FUNCTION "FC_PROG_FSH_OFF" : VOID
TITLE =FC PROG BASE FLASH-OFF
{ S7_language := '9(1) Angielski (Stany Zjednoczone)  11.01.2022  09:45:15' }
VERSION : 0.1

BEGIN
NETWORK
TITLE =

NETWORK
TITLE =Status Flash-Off ON
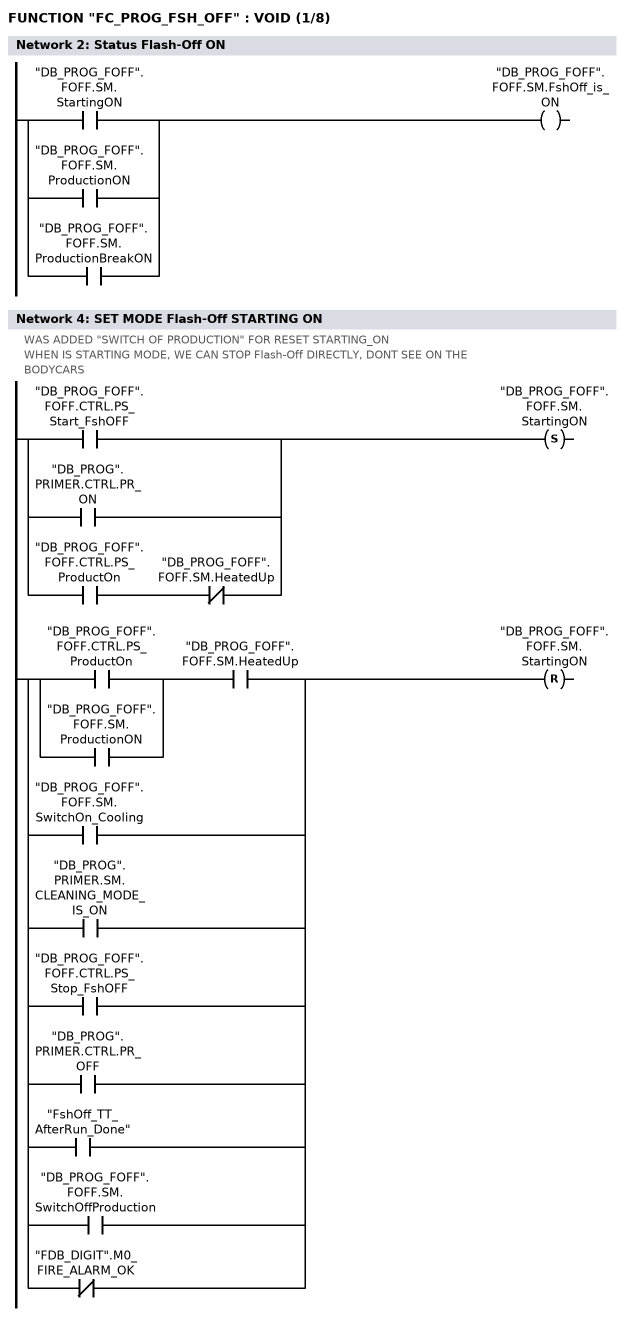
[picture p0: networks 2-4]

      O     "DB_PROG_FOFF".FOFF.SM.StartingON;
      O     "DB_PROG_FOFF".FOFF.SM.ProductionON;
      O     "DB_PROG_FOFF".FOFF.SM.ProductionBreakON;
      =     "DB_PROG_FOFF".FOFF.SM.FshOff_is_ON;
NETWORK
TITLE =SET MODE OF Flash-Off
//
//**************** SET MODE OF Flash-Off
//****************************************************
//


NETWORK
TITLE =SET MODE Flash-Off STARTING ON
//WAS ADDED "SWITCH OF PRODUCTION" FOR RESET STARTING_ON
//WHEN IS STARTING MODE, WE CAN STOP Flash-Off DIRECTLY, DONT SEE ON THE
//BODYCARS
      U(    ;
      O     "DB_PROG_FOFF".FOFF.CTRL.PS_Start_FshOFF;
      O     "DB_PROG".PRIMER.CTRL.PR_ON;
      O     ;
      U     "DB_PROG_FOFF".FOFF.CTRL.PS_ProductOn;
      UN    "DB_PROG_FOFF".FOFF.SM.HeatedUp;
      )     ;
      S     "DB_PROG_FOFF".FOFF.SM.StartingON;
      U(    ;
      U(    ;
      O     "DB_PROG_FOFF".FOFF.CTRL.PS_ProductOn;
      O     "DB_PROG_FOFF".FOFF.SM.ProductionON;
      )     ;
      U     "DB_PROG_FOFF".FOFF.SM.HeatedUp;
      O     "DB_PROG_FOFF".FOFF.SM.SwitchOn_Cooling;
      O     "DB_PROG".PRIMER.SM.CLEANING_MODE_IS_ON;
      O     "DB_PROG_FOFF".FOFF.CTRL.PS_Stop_FshOFF;
      O     "DB_PROG".PRIMER.CTRL.PR_OFF;
      O     "FshOff_TT_AfterRun_Done";
      O     "DB_PROG_FOFF".FOFF.SM.SwitchOffProduction;
      ON    "FDB_DIGIT".M0_FIRE_ALARM_OK;
      )     ;
      R     "DB_PROG_FOFF".FOFF.SM.StartingON;
      NOP   0;
NETWORK
TITLE =FLASH-OFF BASE PRODUCTION ON
//
//-----------------------------------------------------------------
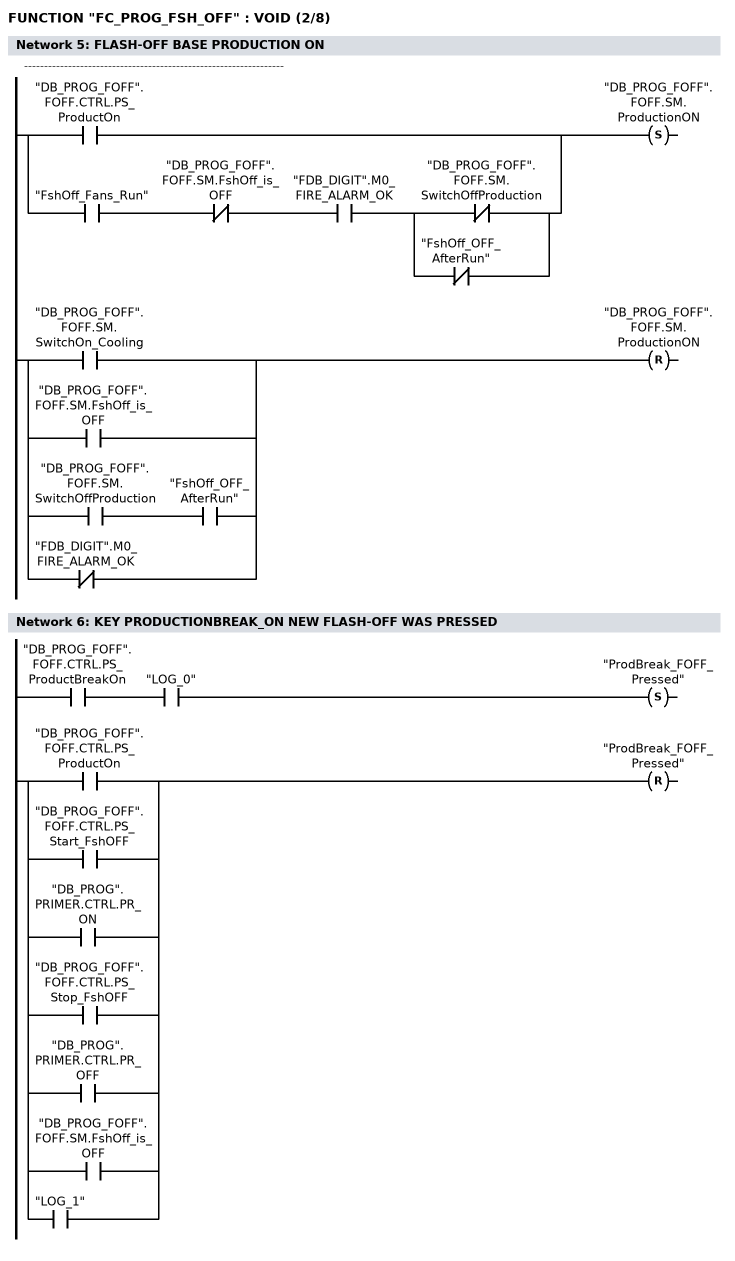
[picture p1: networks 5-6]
      U(    ;
      O     "DB_PROG_FOFF".FOFF.CTRL.PS_ProductOn;
      O     ;
      U     "FshOff_Fans_Run";
      UN    "DB_PROG_FOFF".FOFF.SM.FshOff_is_OFF;
      U     "FDB_DIGIT".M0_FIRE_ALARM_OK;
      U(    ;
      ON    "DB_PROG_FOFF".FOFF.SM.SwitchOffProduction;
      ON    "FshOff_OFF_AfterRun";
      )     ;
      )     ;
      S     "DB_PROG_FOFF".FOFF.SM.ProductionON;
      U(    ;
      O     "DB_PROG_FOFF".FOFF.SM.SwitchOn_Cooling;
      O     "DB_PROG_FOFF".FOFF.SM.FshOff_is_OFF;
      O     ;
      U     "DB_PROG_FOFF".FOFF.SM.SwitchOffProduction;
      U     "FshOff_OFF_AfterRun";
      ON    "FDB_DIGIT".M0_FIRE_ALARM_OK;
      )     ;
      R     "DB_PROG_FOFF".FOFF.SM.ProductionON;
      NOP   0;
NETWORK
TITLE =KEY PRODUCTIONBREAK_ON NEW FLASH-OFF WAS PRESSED

      U     "DB_PROG_FOFF".FOFF.CTRL.PS_ProductBreakOn;
      U     "LOG_0";
      S     "ProdBreak_FOFF_Pressed";
      U(    ;
      O     "DB_PROG_FOFF".FOFF.CTRL.PS_ProductOn;
      O     "DB_PROG_FOFF".FOFF.CTRL.PS_Start_FshOFF;
      O     "DB_PROG".PRIMER.CTRL.PR_ON;
      O     "DB_PROG_FOFF".FOFF.CTRL.PS_Stop_FshOFF;
      O     "DB_PROG".PRIMER.CTRL.PR_OFF;
      O     "DB_PROG_FOFF".FOFF.SM.FshOff_is_OFF;
      O     "LOG_1";
      )     ;
      R     "ProdBreak_FOFF_Pressed";
      NOP   0;
NETWORK
TITLE =SET MODE Flash-Off PRODUCTION BREAK ON
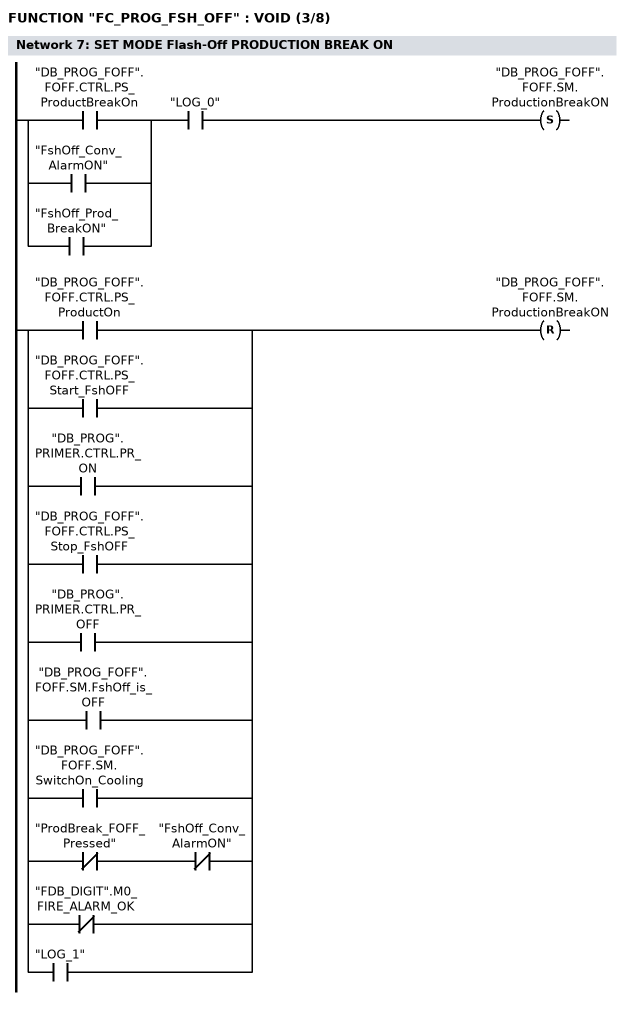
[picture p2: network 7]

      U(    ;
      O     "DB_PROG_FOFF".FOFF.CTRL.PS_ProductBreakOn;
      O     "FshOff_Conv_AlarmON";
      O     "FshOff_Prod_BreakON";
      )     ;
      U     "LOG_0";
      S     "DB_PROG_FOFF".FOFF.SM.ProductionBreakON;
      U(    ;
      O     "DB_PROG_FOFF".FOFF.CTRL.PS_ProductOn;
      O     "DB_PROG_FOFF".FOFF.CTRL.PS_Start_FshOFF;
      O     "DB_PROG".PRIMER.CTRL.PR_ON;
      O     "DB_PROG_FOFF".FOFF.CTRL.PS_Stop_FshOFF;
      O     "DB_PROG".PRIMER.CTRL.PR_OFF;
      O     "DB_PROG_FOFF".FOFF.SM.FshOff_is_OFF;
      O     "DB_PROG_FOFF".FOFF.SM.SwitchOn_Cooling;
      O     ;
      UN    "ProdBreak_FOFF_Pressed";
      UN    "FshOff_Conv_AlarmON";
      ON    "FDB_DIGIT".M0_FIRE_ALARM_OK;
      O     "LOG_1";
      )     ;
      R     "DB_PROG_FOFF".FOFF.SM.ProductionBreakON;
      NOP   0;
NETWORK
TITLE =SET MODE Flash-Off OFF
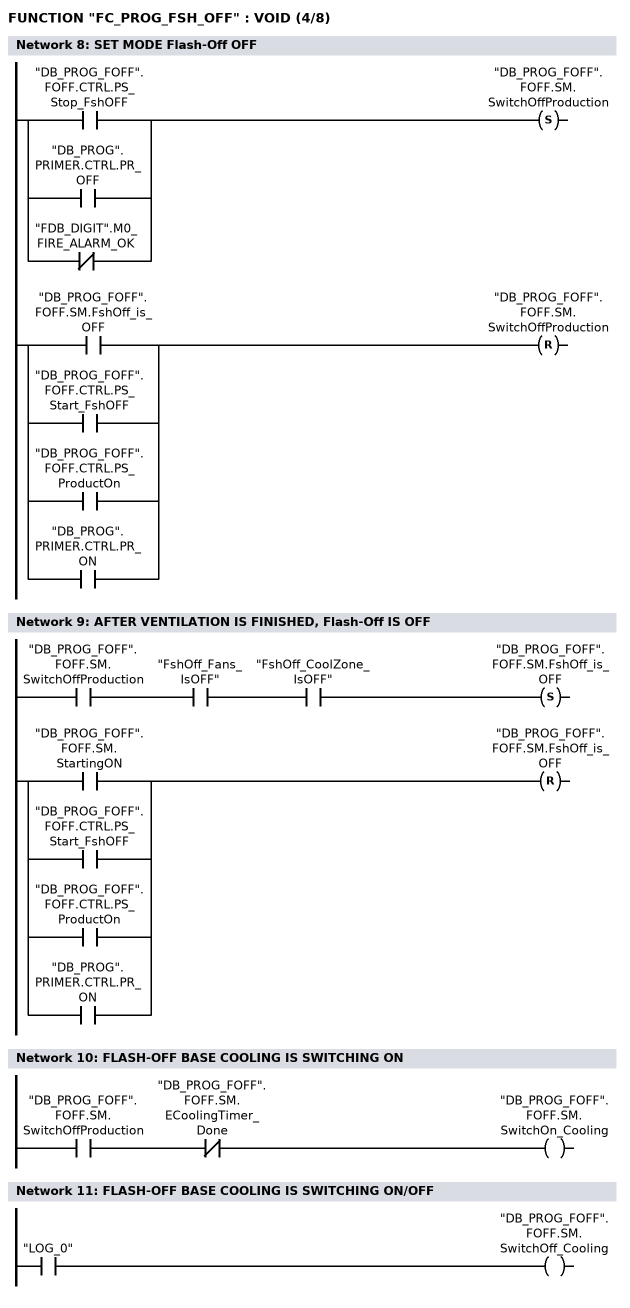
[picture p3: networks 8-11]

      U(    ;
      O     "DB_PROG_FOFF".FOFF.CTRL.PS_Stop_FshOFF;
      O     "DB_PROG".PRIMER.CTRL.PR_OFF;
      ON    "FDB_DIGIT".M0_FIRE_ALARM_OK;
      )     ;
      S     "DB_PROG_FOFF".FOFF.SM.SwitchOffProduction;
      U(    ;
      O     "DB_PROG_FOFF".FOFF.SM.FshOff_is_OFF;
      O     "DB_PROG_FOFF".FOFF.CTRL.PS_Start_FshOFF;
      O     "DB_PROG_FOFF".FOFF.CTRL.PS_ProductOn;
      O     "DB_PROG".PRIMER.CTRL.PR_ON;
      )     ;
      R     "DB_PROG_FOFF".FOFF.SM.SwitchOffProduction;
      NOP   0;
NETWORK
TITLE =AFTER VENTILATION IS FINISHED, Flash-Off IS OFF

      U     "DB_PROG_FOFF".FOFF.SM.SwitchOffProduction;
      U     "FshOff_Fans_IsOFF";
      U     "FshOff_CoolZone_IsOFF";
      S     "DB_PROG_FOFF".FOFF.SM.FshOff_is_OFF;
      U(    ;
      O     "DB_PROG_FOFF".FOFF.SM.StartingON;
      O     "DB_PROG_FOFF".FOFF.CTRL.PS_Start_FshOFF;
      O     "DB_PROG_FOFF".FOFF.CTRL.PS_ProductOn;
      O     "DB_PROG".PRIMER.CTRL.PR_ON;
      )     ;
      R     "DB_PROG_FOFF".FOFF.SM.FshOff_is_OFF;
      NOP   0;
NETWORK
TITLE =FLASH-OFF BASE COOLING IS SWITCHING ON

      U     "DB_PROG_FOFF".FOFF.SM.SwitchOffProduction;
      UN    "DB_PROG_FOFF".FOFF.SM.ECoolingTimer_Done;
      =     "DB_PROG_FOFF".FOFF.SM.SwitchOn_Cooling;
NETWORK
TITLE =FLASH-OFF BASE COOLING IS SWITCHING ON/OFF

      U     "LOG_0";
      =     "DB_PROG_FOFF".FOFF.SM.SwitchOff_Cooling;
NETWORK
TITLE =EMERGENCY COOLING ON
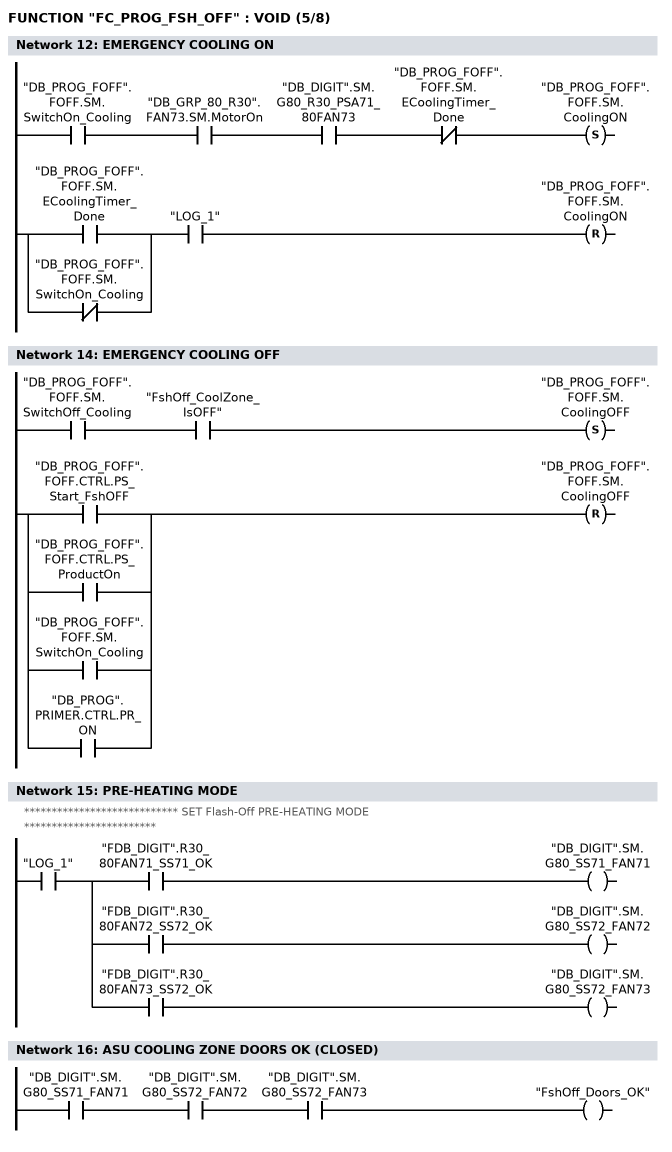
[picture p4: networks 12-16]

      U     "DB_PROG_FOFF".FOFF.SM.SwitchOn_Cooling;
      U     "DB_GRP_80_R30".FAN73.SM.MotorOn;
      U     "DB_DIGIT".SM.G80_R30_PSA71_80FAN73;
      UN    "DB_PROG_FOFF".FOFF.SM.ECoolingTimer_Done;
      S     "DB_PROG_FOFF".FOFF.SM.CoolingON;
      U(    ;
      O     "DB_PROG_FOFF".FOFF.SM.ECoolingTimer_Done;
      ON    "DB_PROG_FOFF".FOFF.SM.SwitchOn_Cooling;
      )     ;
      U     "LOG_1";
      R     "DB_PROG_FOFF".FOFF.SM.CoolingON;
      NOP   0;
NETWORK
TITLE =

NETWORK
TITLE =EMERGENCY COOLING OFF

      U     "DB_PROG_FOFF".FOFF.SM.SwitchOff_Cooling;
      U     "FshOff_CoolZone_IsOFF";
      S     "DB_PROG_FOFF".FOFF.SM.CoolingOFF;
      U(    ;
      O     "DB_PROG_FOFF".FOFF.CTRL.PS_Start_FshOFF;
      O     "DB_PROG_FOFF".FOFF.CTRL.PS_ProductOn;
      O     "DB_PROG_FOFF".FOFF.SM.SwitchOn_Cooling;
      O     "DB_PROG".PRIMER.CTRL.PR_ON;
      )     ;
      R     "DB_PROG_FOFF".FOFF.SM.CoolingOFF;
      NOP   0;
NETWORK
TITLE =PRE-HEATING MODE
//
//**************************** SET Flash-Off PRE-HEATING MODE
//************************
//


      U     "LOG_1";
      =     L      0.0;
      U     L      0.0;
      U     "FDB_DIGIT".R30_80FAN71_SS71_OK;
      =     "DB_DIGIT".SM.G80_SS71_FAN71;
      U     L      0.0;
      U     "FDB_DIGIT".R30_80FAN72_SS72_OK;
      =     "DB_DIGIT".SM.G80_SS72_FAN72;
      U     L      0.0;
      U     "FDB_DIGIT".R30_80FAN73_SS72_OK;
      =     "DB_DIGIT".SM.G80_SS72_FAN73;
NETWORK
TITLE =ASU COOLING ZONE DOORS OK (CLOSED)

      U     "DB_DIGIT".SM.G80_SS71_FAN71;
      U     "DB_DIGIT".SM.G80_SS72_FAN72;
      U     "DB_DIGIT".SM.G80_SS72_FAN73;
      =     "FshOff_Doors_OK";
NETWORK
TITLE =Flash-Off CHAIN ON
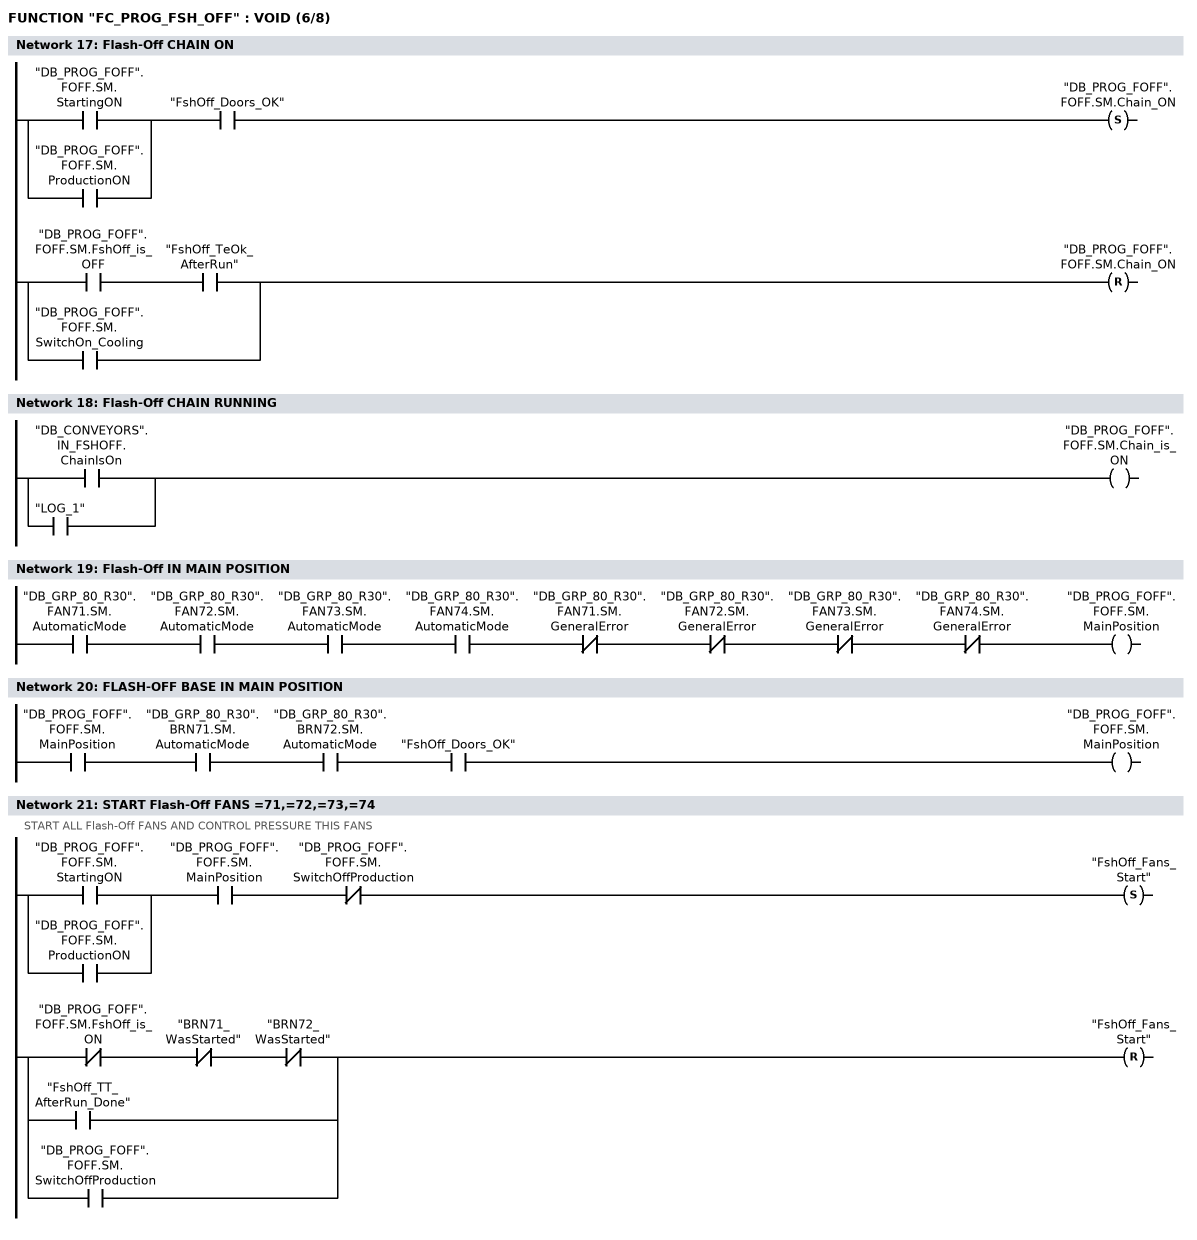
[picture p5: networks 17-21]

      U(    ;
      O     "DB_PROG_FOFF".FOFF.SM.StartingON;
      O     "DB_PROG_FOFF".FOFF.SM.ProductionON;
      )     ;
      U     "FshOff_Doors_OK";
      S     "DB_PROG_FOFF".FOFF.SM.Chain_ON;
      U(    ;
      U     "DB_PROG_FOFF".FOFF.SM.FshOff_is_OFF;
      U     "FshOff_TeOk_AfterRun";
      O     "DB_PROG_FOFF".FOFF.SM.SwitchOn_Cooling;
      )     ;
      R     "DB_PROG_FOFF".FOFF.SM.Chain_ON;
      NOP   0;
NETWORK
TITLE =Flash-Off CHAIN RUNNING

      O     "DB_CONVEYORS".IN_FSHOFF.ChainIsOn;
      O     "LOG_1";
      =     "DB_PROG_FOFF".FOFF.SM.Chain_is_ON;
NETWORK
TITLE =Flash-Off IN MAIN POSITION

      U     "DB_GRP_80_R30".FAN71.SM.AutomaticMode;
      U     "DB_GRP_80_R30".FAN72.SM.AutomaticMode;
      U     "DB_GRP_80_R30".FAN73.SM.AutomaticMode;
      U     "DB_GRP_80_R30".FAN74.SM.AutomaticMode;
      UN    "DB_GRP_80_R30".FAN71.SM.GeneralError;
      UN    "DB_GRP_80_R30".FAN72.SM.GeneralError;
      UN    "DB_GRP_80_R30".FAN73.SM.GeneralError;
      UN    "DB_GRP_80_R30".FAN74.SM.GeneralError;
      =     "DB_PROG_FOFF".FOFF.SM.MainPosition;
NETWORK
TITLE =FLASH-OFF BASE IN MAIN POSITION

      U     "DB_PROG_FOFF".FOFF.SM.MainPosition;
      U     "DB_GRP_80_R30".BRN71.SM.AutomaticMode;
      U     "DB_GRP_80_R30".BRN72.SM.AutomaticMode;
      U     "FshOff_Doors_OK";
      =     "DB_PROG_FOFF".FOFF.SM.MainPosition;
NETWORK
TITLE =START Flash-Off FANS =71,=72,=73,=74
//START ALL Flash-Off FANS AND CONTROL PRESSURE THIS FANS
//
//
      U(    ;
      O     "DB_PROG_FOFF".FOFF.SM.StartingON;
      O     "DB_PROG_FOFF".FOFF.SM.ProductionON;
      )     ;
      U     "DB_PROG_FOFF".FOFF.SM.MainPosition;
      UN    "DB_PROG_FOFF".FOFF.SM.SwitchOffProduction;
      S     "FshOff_Fans_Start";
      U(    ;
      UN    "DB_PROG_FOFF".FOFF.SM.FshOff_is_ON;
      UN    "BRN71_WasStarted";
      UN    "BRN72_WasStarted";
      O     "FshOff_TT_AfterRun_Done";
      O     "DB_PROG_FOFF".FOFF.SM.SwitchOffProduction;
      )     ;
      R     "FshOff_Fans_Start";
      NOP   0;
NETWORK
TITLE =
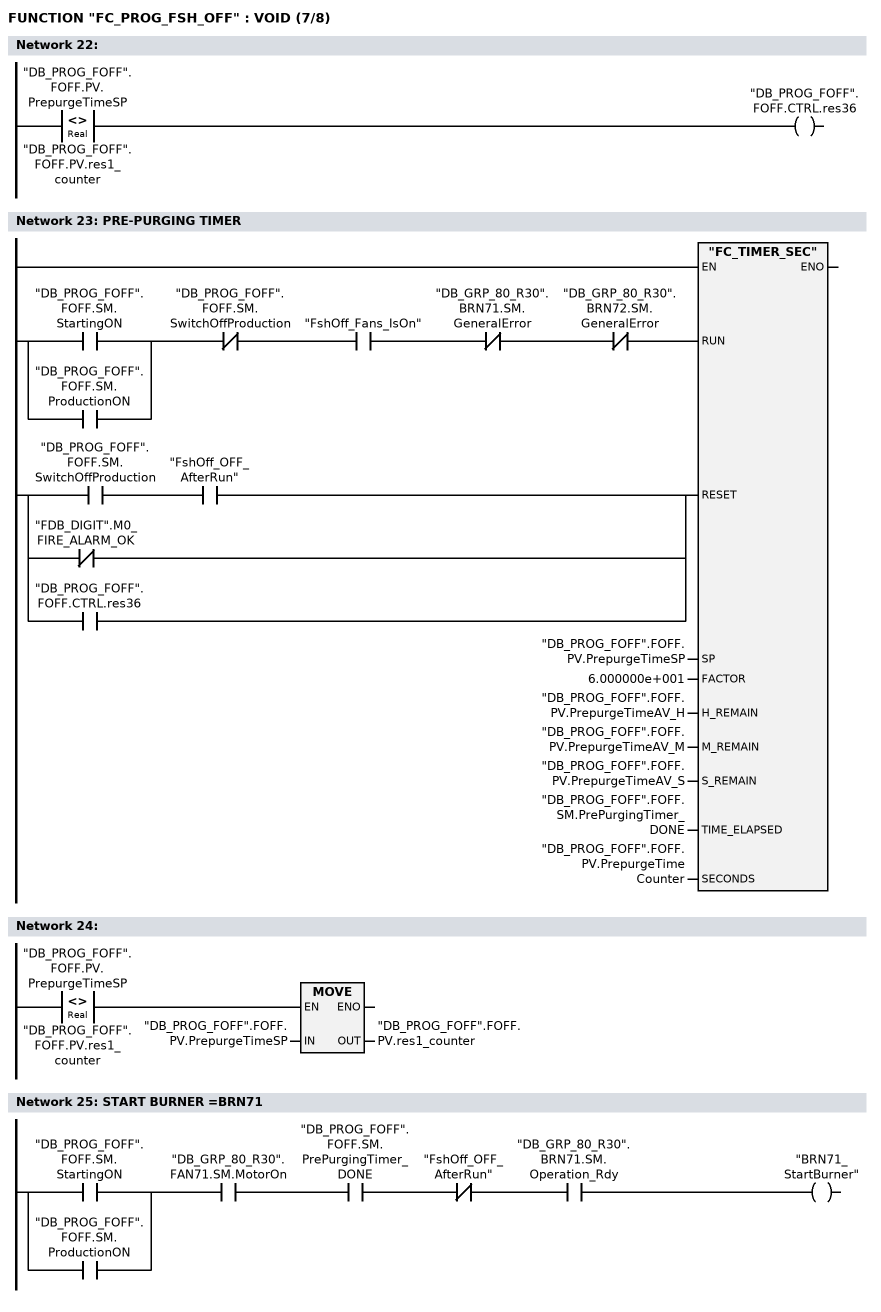
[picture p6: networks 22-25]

      L     "DB_PROG_FOFF".FOFF.PV.PrepurgeTimeSP;
      L     "DB_PROG_FOFF".FOFF.PV.res1_counter;
      <>R   ;
      =     "DB_PROG_FOFF".FOFF.CTRL.res36;
NETWORK
TITLE =PRE-PURGING TIMER

      U(    ;
      O     "DB_PROG_FOFF".FOFF.SM.StartingON;
      O     "DB_PROG_FOFF".FOFF.SM.ProductionON;
      )     ;
      UN    "DB_PROG_FOFF".FOFF.SM.SwitchOffProduction;
      U     "FshOff_Fans_IsOn";
      UN    "DB_GRP_80_R30".BRN71.SM.GeneralError;
      UN    "DB_GRP_80_R30".BRN72.SM.GeneralError;
      =     L      0.0;
      BLD   103;
      U(    ;
      U     "DB_PROG_FOFF".FOFF.SM.SwitchOffProduction;
      U     "FshOff_OFF_AfterRun";
      ON    "FDB_DIGIT".M0_FIRE_ALARM_OK;
      O     "DB_PROG_FOFF".FOFF.CTRL.res36;
      )     ;
      =     L      0.1;
      BLD   103;
      CALL "FC_TIMER_SEC" (
           RUN                      := L      0.0,
           RESET                    := L      0.1,
           SP                       := "DB_PROG_FOFF".FOFF.PV.PrepurgeTimeSP,
           FACTOR                   := 6.000000e+001,
           H_REMAIN                 := "DB_PROG_FOFF".FOFF.PV.PrepurgeTimeAV_H,
           M_REMAIN                 := "DB_PROG_FOFF".FOFF.PV.PrepurgeTimeAV_M,
           S_REMAIN                 := "DB_PROG_FOFF".FOFF.PV.PrepurgeTimeAV_S,
           TIME_ELAPSED             := "DB_PROG_FOFF".FOFF.SM.PrePurgingTimer_DONE,
           SECONDS                  := "DB_PROG_FOFF".FOFF.PV.PrepurgeTimeCounter);
      NOP   0;
NETWORK
TITLE =

      U(    ;
      L     "DB_PROG_FOFF".FOFF.PV.PrepurgeTimeSP;
      L     "DB_PROG_FOFF".FOFF.PV.res1_counter;
      <>R   ;
      )     ;
      SPBNB _001;
      L     "DB_PROG_FOFF".FOFF.PV.PrepurgeTimeSP;
      T     "DB_PROG_FOFF".FOFF.PV.res1_counter;
_001: NOP   0;
NETWORK
TITLE =START BURNER =BRN71

      U(    ;
      O     "DB_PROG_FOFF".FOFF.SM.StartingON;
      O     "DB_PROG_FOFF".FOFF.SM.ProductionON;
      )     ;
      U     "DB_GRP_80_R30".FAN71.SM.MotorOn;
      U     "DB_PROG_FOFF".FOFF.SM.PrePurgingTimer_DONE;
      UN    "FshOff_OFF_AfterRun";
      U     "DB_GRP_80_R30".BRN71.SM.Operation_Rdy;
      =     "BRN71_StartBurner";
NETWORK
TITLE =START BURNER =BRN72
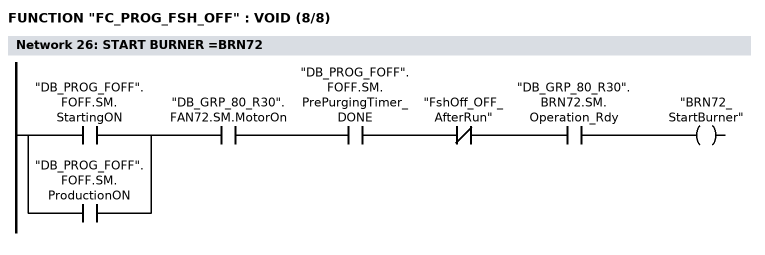
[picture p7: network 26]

      U(    ;
      O     "DB_PROG_FOFF".FOFF.SM.StartingON;
      O     "DB_PROG_FOFF".FOFF.SM.ProductionON;
      )     ;
      U     "DB_GRP_80_R30".FAN72.SM.MotorOn;
      U     "DB_PROG_FOFF".FOFF.SM.PrePurgingTimer_DONE;
      UN    "FshOff_OFF_AfterRun";
      U     "DB_GRP_80_R30".BRN72.SM.Operation_Rdy;
      =     "BRN72_StartBurner";
NETWORK
TITLE =

      U     "LOG_1";
      =     L      0.0;
      U     L      0.0;
      U(    ;
      L     "DB_GRP_80_R30".TIC71_IN_GR1.PV.SP_AV;
      L     0.000000e+000;
      <=R   ;
      )     ;
      SPBNB _002;
      L     6.000000e+001;
      T     "DB_GRP_80_R30".TIC71_IN_GR1.PV.SP_AV;
_002: NOP   0;
      U(    ;
      U     L      0.0;
      SPBNB _003;
      L     "DB_GRP_80_R30".TIC71_IN_GR1.PV.SP_AV;
      L     5.000000e+000;
      -R    ;
      T     "DB_GRP_80_R30".TIC71_IN_GR1.PV.Limit_01;
      UN    OV;
      SAVE  ;
      CLR   ;
_003: U     BIE;
      )     ;
      SPBNB _004;
      L     "DB_GRP_80_R30".TIC71_IN_GR1.PV.SP_AV;
      L     5.000000e+000;
      +R    ;
      T     "DB_GRP_80_R30".TIC71_IN_GR1.PV.Limit_04;
_004: NOP   0;
NETWORK
TITLE =

      U     "LOG_1";
      =     L      0.0;
      U     L      0.0;
      U(    ;
      L     "DB_GRP_80_R30".TIC71_IN_GR2.PV.SP_AV;
      L     0.000000e+000;
      <=R   ;
      )     ;
      SPBNB _005;
      L     6.000000e+001;
      T     "DB_GRP_80_R30".TIC71_IN_GR2.PV.SP_AV;
_005: NOP   0;
      U(    ;
      U     L      0.0;
      SPBNB _006;
      L     "DB_GRP_80_R30".TIC71_IN_GR2.PV.SP_AV;
      L     5.000000e+000;
      -R    ;
      T     "DB_GRP_80_R30".TIC71_IN_GR2.PV.Limit_01;
      UN    OV;
      SAVE  ;
      CLR   ;
_006: U     BIE;
      )     ;
      SPBNB _007;
      L     "DB_GRP_80_R30".TIC71_IN_GR2.PV.SP_AV;
      L     5.000000e+000;
      +R    ;
      T     "DB_GRP_80_R30".TIC71_IN_GR2.PV.Limit_04;
_007: NOP   0;
NETWORK
TITLE =

      U     "LOG_1";
      =     L      0.0;
      U     L      0.0;
      U(    ;
      L     "DB_GRP_80_R30".TIC75_IN_COOL.PV.SP_AV;
      L     0.000000e+000;
      <=R   ;
      )     ;
      SPBNB _008;
      L     2.000000e+001;
      T     "DB_GRP_80_R30".TIC75_IN_COOL.PV.SP_AV;
_008: NOP   0;
      U(    ;
      U     L      0.0;
      SPBNB _009;
      L     "DB_GRP_80_R30".TIC75_IN_COOL.PV.SP_AV;
      L     5.000000e+000;
      -R    ;
      T     "DB_GRP_80_R30".TIC75_IN_COOL.PV.Limit_01;
      UN    OV;
      SAVE  ;
      CLR   ;
_009: U     BIE;
      )     ;
      SPBNB _00a;
      L     "DB_GRP_80_R30".TIC75_IN_COOL.PV.SP_AV;
      L     5.000000e+000;
      +R    ;
      T     "DB_GRP_80_R30".TIC75_IN_COOL.PV.Limit_04;
_00a: NOP   0;
NETWORK
TITLE =Flash-Off GROUP =71/=72/ TEMPERATURE OK
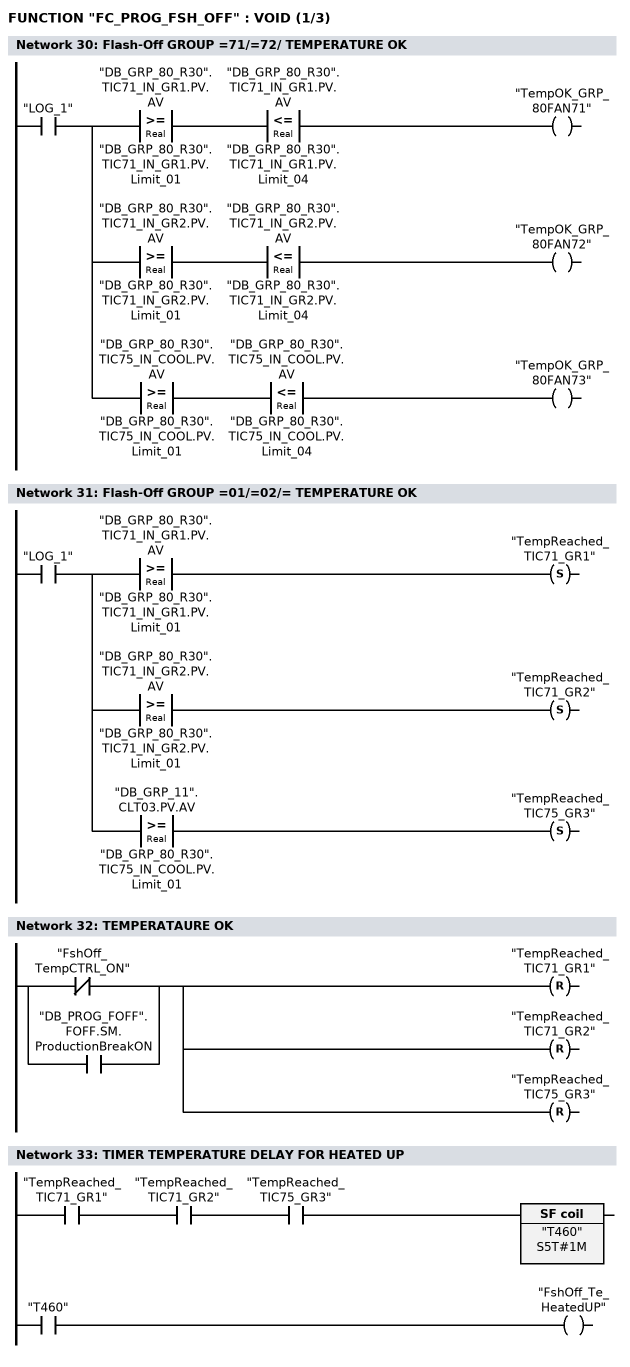
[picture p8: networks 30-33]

      U     "LOG_1";
      =     L      0.0;
      U     L      0.0;
      U(    ;
      L     "DB_GRP_80_R30".TIC71_IN_GR1.PV.AV;
      L     "DB_GRP_80_R30".TIC71_IN_GR1.PV.Limit_01;
      >=R   ;
      )     ;
      U(    ;
      L     "DB_GRP_80_R30".TIC71_IN_GR1.PV.AV;
      L     "DB_GRP_80_R30".TIC71_IN_GR1.PV.Limit_04;
      <=R   ;
      )     ;
      =     "TempOK_GRP_80FAN71";
      U     L      0.0;
      U(    ;
      L     "DB_GRP_80_R30".TIC71_IN_GR2.PV.AV;
      L     "DB_GRP_80_R30".TIC71_IN_GR2.PV.Limit_01;
      >=R   ;
      )     ;
      U(    ;
      L     "DB_GRP_80_R30".TIC71_IN_GR2.PV.AV;
      L     "DB_GRP_80_R30".TIC71_IN_GR2.PV.Limit_04;
      <=R   ;
      )     ;
      =     "TempOK_GRP_80FAN72";
      U     L      0.0;
      U(    ;
      L     "DB_GRP_80_R30".TIC75_IN_COOL.PV.AV;
      L     "DB_GRP_80_R30".TIC75_IN_COOL.PV.Limit_01;
      >=R   ;
      )     ;
      U(    ;
      L     "DB_GRP_80_R30".TIC75_IN_COOL.PV.AV;
      L     "DB_GRP_80_R30".TIC75_IN_COOL.PV.Limit_04;
      <=R   ;
      )     ;
      =     "TempOK_GRP_80FAN73";
NETWORK
TITLE =Flash-Off GROUP =01/=02/= TEMPERATURE OK

      U     "LOG_1";
      =     L      0.0;
      U     L      0.0;
      U(    ;
      L     "DB_GRP_80_R30".TIC71_IN_GR1.PV.AV;
      L     "DB_GRP_80_R30".TIC71_IN_GR1.PV.Limit_01;
      >=R   ;
      )     ;
      S     "TempReached_TIC71_GR1";
      U     L      0.0;
      U(    ;
      L     "DB_GRP_80_R30".TIC71_IN_GR2.PV.AV;
      L     "DB_GRP_80_R30".TIC71_IN_GR2.PV.Limit_01;
      >=R   ;
      )     ;
      S     "TempReached_TIC71_GR2";
      U     L      0.0;
      U(    ;
      L     "DB_GRP_11".CLT03.PV.AV;
      L     "DB_GRP_80_R30".TIC75_IN_COOL.PV.Limit_01;
      >=R   ;
      )     ;
      S     "TempReached_TIC75_GR3";
NETWORK
TITLE =TEMPERATAURE OK

      ON    "FshOff_TempCTRL_ON";
      O     "DB_PROG_FOFF".FOFF.SM.ProductionBreakON;
      R     "TempReached_TIC71_GR1";
      R     "TempReached_TIC71_GR2";
      R     "TempReached_TIC75_GR3";
NETWORK
TITLE =TIMER TEMPERATURE DELAY FOR HEATED UP

      U     "TempReached_TIC71_GR1";
      U     "TempReached_TIC71_GR2";
      U     "TempReached_TIC75_GR3";
      L     S5T#1M;
      SA    "T460";
      NOP   0;
      NOP   0;
      NOP   0;
      U     "T460";
      =     "FshOff_Te_HeatedUP";
NETWORK
TITLE =ALL HEATING BOXES (Flash-OffS) - TEMPERATURE OK
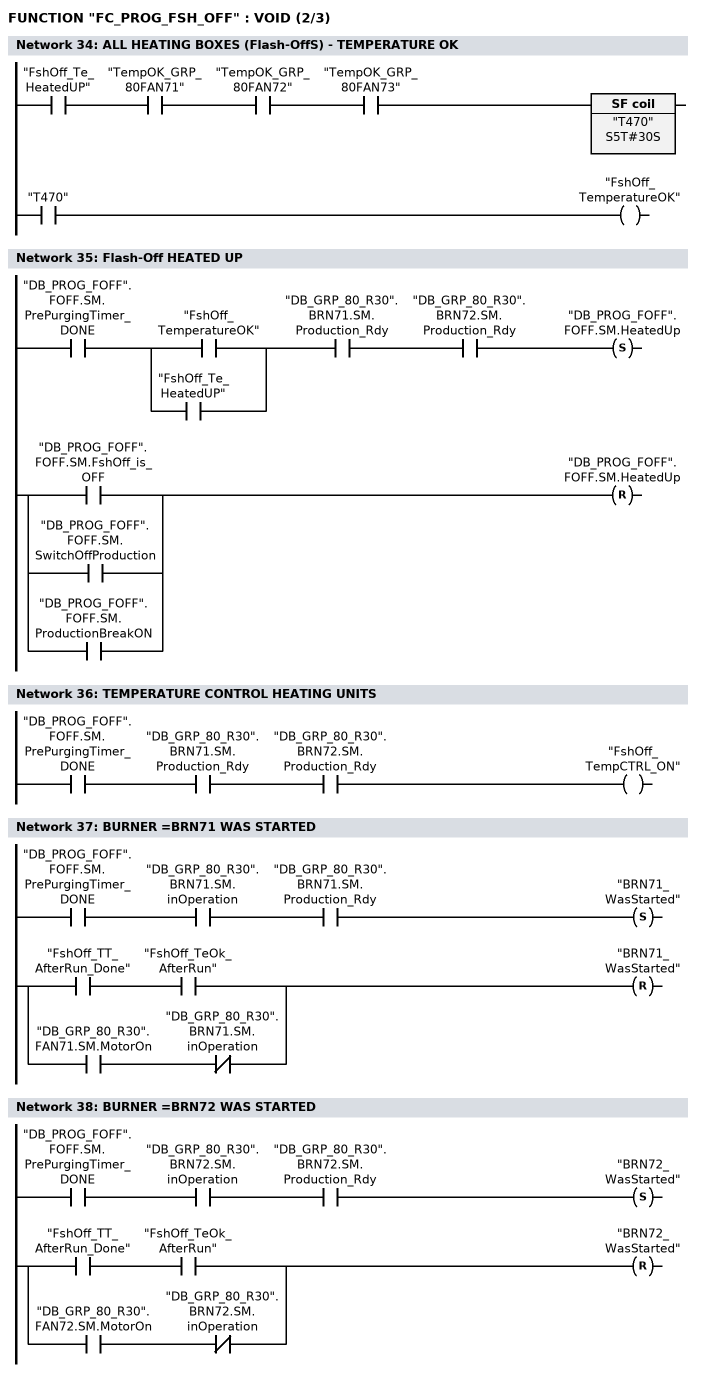
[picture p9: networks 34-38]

      U     "FshOff_Te_HeatedUP";
      U     "TempOK_GRP_80FAN71";
      U     "TempOK_GRP_80FAN72";
      U     "TempOK_GRP_80FAN73";
      L     S5T#30S;
      SA    "T470";
      NOP   0;
      NOP   0;
      NOP   0;
      U     "T470";
      =     "FshOff_TemperatureOK";
NETWORK
TITLE =Flash-Off HEATED UP

      U     "DB_PROG_FOFF".FOFF.SM.PrePurgingTimer_DONE;
      U(    ;
      O     "FshOff_TemperatureOK";
      O     "FshOff_Te_HeatedUP";
      )     ;
      U     "DB_GRP_80_R30".BRN71.SM.Production_Rdy;
      U     "DB_GRP_80_R30".BRN72.SM.Production_Rdy;
      S     "DB_PROG_FOFF".FOFF.SM.HeatedUp;
      U(    ;
      O     "DB_PROG_FOFF".FOFF.SM.FshOff_is_OFF;
      O     "DB_PROG_FOFF".FOFF.SM.SwitchOffProduction;
      O     "DB_PROG_FOFF".FOFF.SM.ProductionBreakON;
      )     ;
      R     "DB_PROG_FOFF".FOFF.SM.HeatedUp;
      NOP   0;
NETWORK
TITLE =TEMPERATURE CONTROL HEATING UNITS

      U     "DB_PROG_FOFF".FOFF.SM.PrePurgingTimer_DONE;
      U     "DB_GRP_80_R30".BRN71.SM.Production_Rdy;
      U     "DB_GRP_80_R30".BRN72.SM.Production_Rdy;
      =     "FshOff_TempCTRL_ON";
NETWORK
TITLE =BURNER =BRN71 WAS STARTED

      U     "DB_PROG_FOFF".FOFF.SM.PrePurgingTimer_DONE;
      U     "DB_GRP_80_R30".BRN71.SM.inOperation;
      U     "DB_GRP_80_R30".BRN71.SM.Production_Rdy;
      S     "BRN71_WasStarted";
      U(    ;
      U     "FshOff_TT_AfterRun_Done";
      U     "FshOff_TeOk_AfterRun";
      O     ;
      U     "DB_GRP_80_R30".FAN71.SM.MotorOn;
      UN    "DB_GRP_80_R30".BRN71.SM.inOperation;
      )     ;
      R     "BRN71_WasStarted";
      NOP   0;
NETWORK
TITLE =BURNER =BRN72 WAS STARTED

      U     "DB_PROG_FOFF".FOFF.SM.PrePurgingTimer_DONE;
      U     "DB_GRP_80_R30".BRN72.SM.inOperation;
      U     "DB_GRP_80_R30".BRN72.SM.Production_Rdy;
      S     "BRN72_WasStarted";
      U(    ;
      U     "FshOff_TT_AfterRun_Done";
      U     "FshOff_TeOk_AfterRun";
      O     ;
      U     "DB_GRP_80_R30".FAN72.SM.MotorOn;
      UN    "DB_GRP_80_R30".BRN72.SM.inOperation;
      )     ;
      R     "BRN72_WasStarted";
      NOP   0;
NETWORK
TITLE =FLASH-OFF BASE RELEASE FOR OPERATION
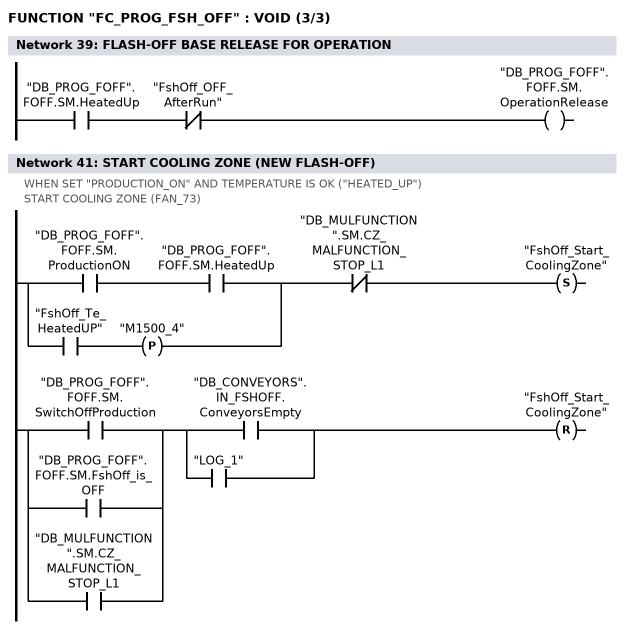
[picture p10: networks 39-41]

      U     "DB_PROG_FOFF".FOFF.SM.HeatedUp;
      UN    "FshOff_OFF_AfterRun";
      =     "DB_PROG_FOFF".FOFF.SM.OperationRelease;
NETWORK
TITLE =PRODUCTION MODE
//
//******************** SET Flash-Off PRODUCTION MODE
//*************************************************************************
//
NETWORK
TITLE =START COOLING ZONE (NEW FLASH-OFF)
//WHEN SET "PRODUCTION_ON" AND TEMPERATURE IS OK ("HEATED_UP")
//START COOLING ZONE (FAN_73)
      U(    ;
      U     "DB_PROG_FOFF".FOFF.SM.ProductionON;
      U     "DB_PROG_FOFF".FOFF.SM.HeatedUp;
      O(    ;
      U     "FshOff_Te_HeatedUP";
      FP    "M1500_4";
      )     ;
      )     ;
      UN    "DB_MULFUNCTION".SM.CZ_MALFUNCTION_STOP_L1;
      S     "FshOff_Start_CoolingZone";
      U(    ;
      O     "DB_PROG_FOFF".FOFF.SM.SwitchOffProduction;
      O     "DB_PROG_FOFF".FOFF.SM.FshOff_is_OFF;
      O     "DB_MULFUNCTION".SM.CZ_MALFUNCTION_STOP_L1;
      )     ;
      U(    ;
      O     "DB_CONVEYORS".IN_FSHOFF.ConveyorsEmpty;
      O     "LOG_1";
      )     ;
      R     "FshOff_Start_CoolingZone";
      NOP   0;
NETWORK
TITLE =



NETWORK
TITLE =TIMER PAUSE TO START SUPPLY AIR FAN =80FANxxx_M1
//WHEN SYSTEMS ARE IN MAIN (START) CONDITION,
//SET TIMER DELAY AND START AIR FANS
//---------------------------------------------------------------
//Step 1
//
//1° =80FAN71;
//2° =80FAN72;
//AFTER PURGE:
//3° =BURNER;
//4° =DRYER SYSTEM;
//
//Step 2
//1° =80FAN74;
//2° =80FAN73;
//3° =COLD VALVE REGULATION;
//-------------------------
      U     "FshOff_Fans_Start";
      =     L      0.0;
      U     L      0.0;
      L     S5T#1S;
      SE    "T463";
      NOP   0;
      NOP   0;
      NOP   0;
      U     "T463";
      =     "T_80FAN71_DONE";
      U     L      0.0;
      U     "T_80FAN71_DONE";
      U     "DB_GRP_80_R30".FAN71.SM.MotorOn;
      L     S5T#15S;
      SE    "T464";
      NOP   0;
      NOP   0;
      NOP   0;
      U     "T464";
      =     "T_80FAN72_DONE";
      U     L      0.0;
      U     "FshOff_Fans_IsOn";
      =     L      0.1;
      U     L      0.1;
      U(    ;
      O     "BRN71_WasStarted";
      O     "BRN72_WasStarted";
      )     ;
      U(    ;
      O     "FshOff_Start_CoolingZone";
      O     "LOG_1";
      )     ;
      L     S5T#10S;
      SE    "T465";
      NOP   0;
      NOP   0;
      NOP   0;
      U     "T465";
      =     "T_80FAN73_DONE";
      U     L      0.1;
      U     "DB_GRP_80_R30".FAN73.SM.MotorOn;
      L     S5T#10S;
      SE    "T466";
      NOP   0;
      NOP   0;
      NOP   0;
      U     "T466";
      =     "T_80FAN74_DONE";
NETWORK
TITLE =WHEN ALL FANS RUNNING AND PRESSURE SENSORS ARE OK
//WHEN TEMPERATURE IN ALL HEATING BOXES OK, FANS RUNNING AND PRESSURE SENSORS ARE
//OK - SET STATUS "RELEASE OF PRODUCTION Flash-Off" AND "RELEASE FOR CONVEYING"
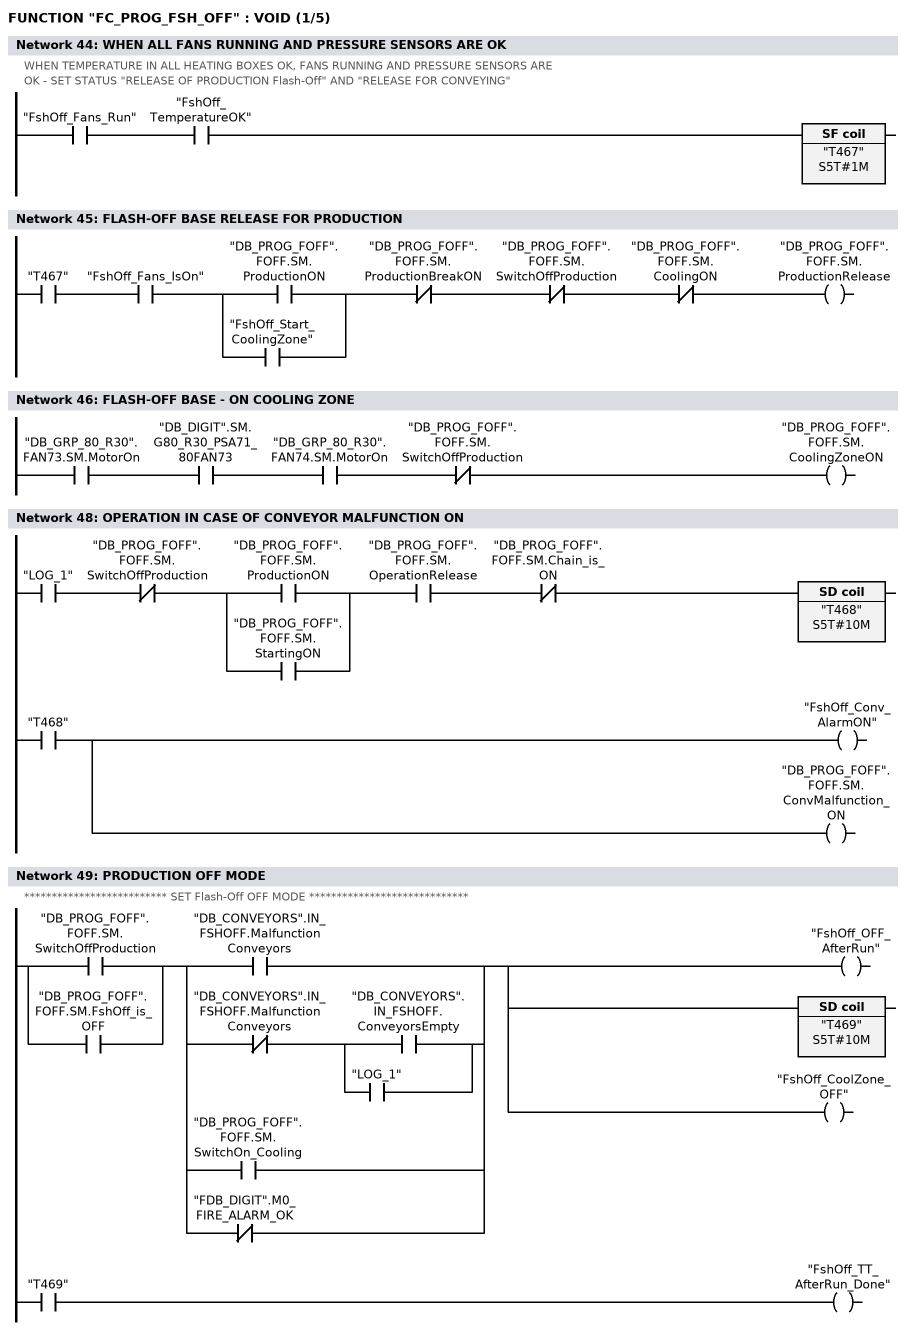
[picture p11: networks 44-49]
      U     "FshOff_Fans_Run";
      U     "FshOff_TemperatureOK";
      L     S5T#1M;
      SA    "T467";
      NOP   0;
      NOP   0;
      NOP   0;
      NOP   0;
NETWORK
TITLE =FLASH-OFF BASE RELEASE FOR PRODUCTION

      U     "T467";
      U     "FshOff_Fans_IsOn";
      U(    ;
      O     "DB_PROG_FOFF".FOFF.SM.ProductionON;
      O     "FshOff_Start_CoolingZone";
      )     ;
      UN    "DB_PROG_FOFF".FOFF.SM.ProductionBreakON;
      UN    "DB_PROG_FOFF".FOFF.SM.SwitchOffProduction;
      UN    "DB_PROG_FOFF".FOFF.SM.CoolingON;
      =     "DB_PROG_FOFF".FOFF.SM.ProductionRelease;
NETWORK
TITLE =FLASH-OFF BASE - ON COOLING ZONE

      U     "DB_GRP_80_R30".FAN73.SM.MotorOn;
      U     "DB_DIGIT".SM.G80_R30_PSA71_80FAN73;
      U     "DB_GRP_80_R30".FAN74.SM.MotorOn;
      UN    "DB_PROG_FOFF".FOFF.SM.SwitchOffProduction;
      =     "DB_PROG_FOFF".FOFF.SM.CoolingZoneON;
NETWORK
TITLE =PRODUCTION BREAK MODE
//
//********************** SET Flash-Off PRODUCTION BREAK MODE
//************************
//


NETWORK
TITLE =OPERATION IN CASE OF CONVEYOR MALFUNCTION ON

      U     "LOG_1";
      UN    "DB_PROG_FOFF".FOFF.SM.SwitchOffProduction;
      U(    ;
      O     "DB_PROG_FOFF".FOFF.SM.ProductionON;
      O     "DB_PROG_FOFF".FOFF.SM.StartingON;
      )     ;
      U     "DB_PROG_FOFF".FOFF.SM.OperationRelease;
      UN    "DB_PROG_FOFF".FOFF.SM.Chain_is_ON;
      L     S5T#10M;
      SE    "T468";
      NOP   0;
      NOP   0;
      NOP   0;
      U     "T468";
      =     "FshOff_Conv_AlarmON";
      =     "DB_PROG_FOFF".FOFF.SM.ConvMalfunction_ON;
NETWORK
TITLE =PRODUCTION OFF MODE
//
//************************** SET Flash-Off OFF MODE *****************************
//
      U(    ;
      O     "DB_PROG_FOFF".FOFF.SM.SwitchOffProduction;
      O     "DB_PROG_FOFF".FOFF.SM.FshOff_is_OFF;
      )     ;
      U(    ;
      O     "DB_CONVEYORS".IN_FSHOFF.MalfunctionConveyors;
      O     ;
      UN    "DB_CONVEYORS".IN_FSHOFF.MalfunctionConveyors;
      U(    ;
      O     "DB_CONVEYORS".IN_FSHOFF.ConveyorsEmpty;
      O     "LOG_1";
      )     ;
      O     "DB_PROG_FOFF".FOFF.SM.SwitchOn_Cooling;
      ON    "FDB_DIGIT".M0_FIRE_ALARM_OK;
      )     ;
      =     L      0.0;
      U     L      0.0;
      BLD   102;
      =     "FshOff_OFF_AfterRun";
      U     L      0.0;
      L     S5T#10M;
      SE    "T469";
      NOP   0;
      NOP   0;
      NOP   0;
      U     "T469";
      =     "FshOff_TT_AfterRun_Done";
      U     L      0.0;
      BLD   102;
      =     "FshOff_CoolZone_OFF";
NETWORK
TITLE =BURNER ZONE FLASH-OFF, TEMPERATURE OK AFTER RUN
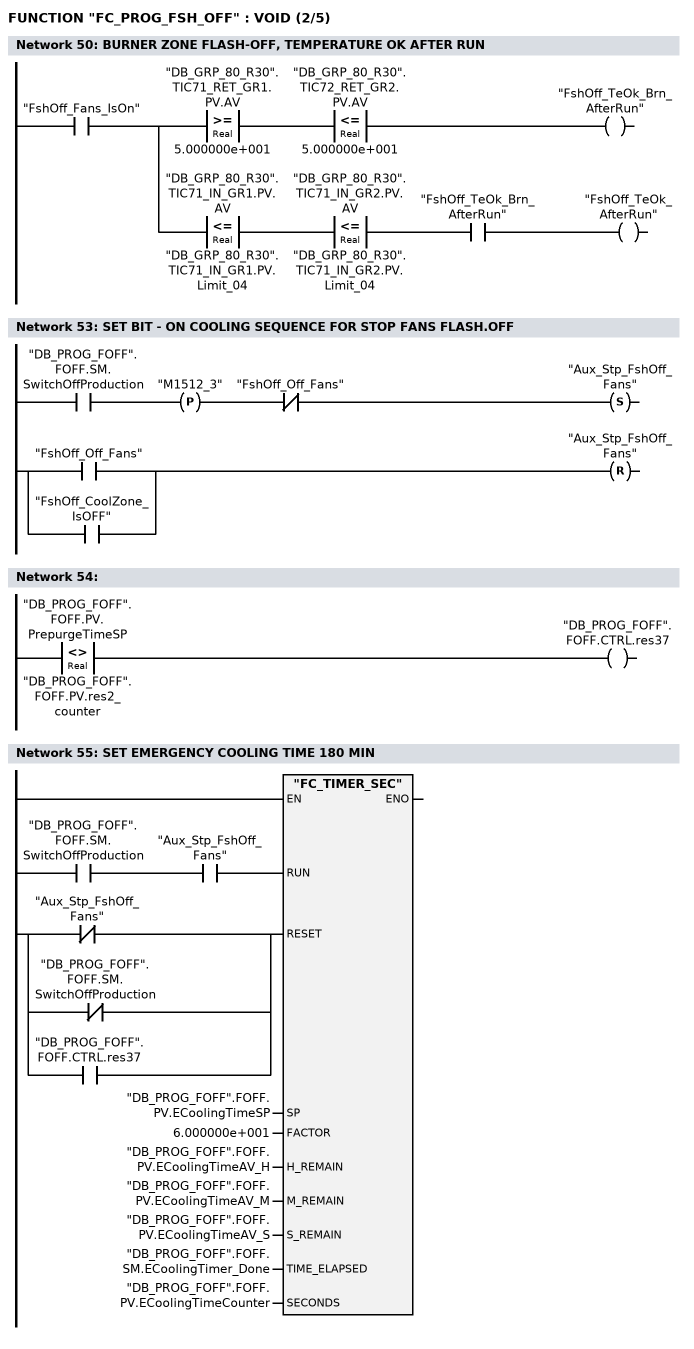
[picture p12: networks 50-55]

      U     "FshOff_Fans_IsOn";
      =     L      0.0;
      U     L      0.0;
      U(    ;
      L     "DB_GRP_80_R30".TIC71_RET_GR1.PV.AV;
      L     5.000000e+001;
      >=R   ;
      )     ;
      U(    ;
      L     "DB_GRP_80_R30".TIC72_RET_GR2.PV.AV;
      L     5.000000e+001;
      <=R   ;
      )     ;
      =     "FshOff_TeOk_Brn_AfterRun";
      U     L      0.0;
      U(    ;
      L     "DB_GRP_80_R30".TIC71_IN_GR1.PV.AV;
      L     "DB_GRP_80_R30".TIC71_IN_GR1.PV.Limit_04;
      <=R   ;
      )     ;
      U(    ;
      L     "DB_GRP_80_R30".TIC71_IN_GR2.PV.AV;
      L     "DB_GRP_80_R30".TIC71_IN_GR2.PV.Limit_04;
      <=R   ;
      )     ;
      U     "FshOff_TeOk_Brn_AfterRun";
      =     "FshOff_TeOk_AfterRun";
NETWORK
TITLE =



NETWORK
TITLE =SET EMERGENCY COOLING MODE
//
//************************ - SET EMERGENCY COOLING MODE - **********************
//


NETWORK
TITLE =SET BIT - ON COOLING SEQUENCE FOR STOP FANS FLASH.OFF

      U     "DB_PROG_FOFF".FOFF.SM.SwitchOffProduction;
      FP    "M1512_3";
      UN    "FshOff_Off_Fans";
      S     "Aux_Stp_FshOff_Fans";
      U(    ;
      O     "FshOff_Off_Fans";
      O     "FshOff_CoolZone_IsOFF";
      )     ;
      R     "Aux_Stp_FshOff_Fans";
      NOP   0;
NETWORK
TITLE =

      L     "DB_PROG_FOFF".FOFF.PV.PrepurgeTimeSP;
      L     "DB_PROG_FOFF".FOFF.PV.res2_counter;
      <>R   ;
      =     "DB_PROG_FOFF".FOFF.CTRL.res37;
NETWORK
TITLE =SET EMERGENCY COOLING TIME 180 MIN

      U     "DB_PROG_FOFF".FOFF.SM.SwitchOffProduction;
      U     "Aux_Stp_FshOff_Fans";
      =     L      0.0;
      BLD   103;
      U(    ;
      ON    "Aux_Stp_FshOff_Fans";
      ON    "DB_PROG_FOFF".FOFF.SM.SwitchOffProduction;
      O     "DB_PROG_FOFF".FOFF.CTRL.res37;
      )     ;
      =     L      0.1;
      BLD   103;
      CALL "FC_TIMER_SEC" (
           RUN                      := L      0.0,
           RESET                    := L      0.1,
           SP                       := "DB_PROG_FOFF".FOFF.PV.ECoolingTimeSP,
           FACTOR                   := 6.000000e+001,
           H_REMAIN                 := "DB_PROG_FOFF".FOFF.PV.ECoolingTimeAV_H,
           M_REMAIN                 := "DB_PROG_FOFF".FOFF.PV.ECoolingTimeAV_M,
           S_REMAIN                 := "DB_PROG_FOFF".FOFF.PV.ECoolingTimeAV_S,
           TIME_ELAPSED             := "DB_PROG_FOFF".FOFF.SM.ECoolingTimer_Done,
           SECONDS                  := "DB_PROG_FOFF".FOFF.PV.ECoolingTimeCounter);
      NOP   0;
NETWORK
TITLE =
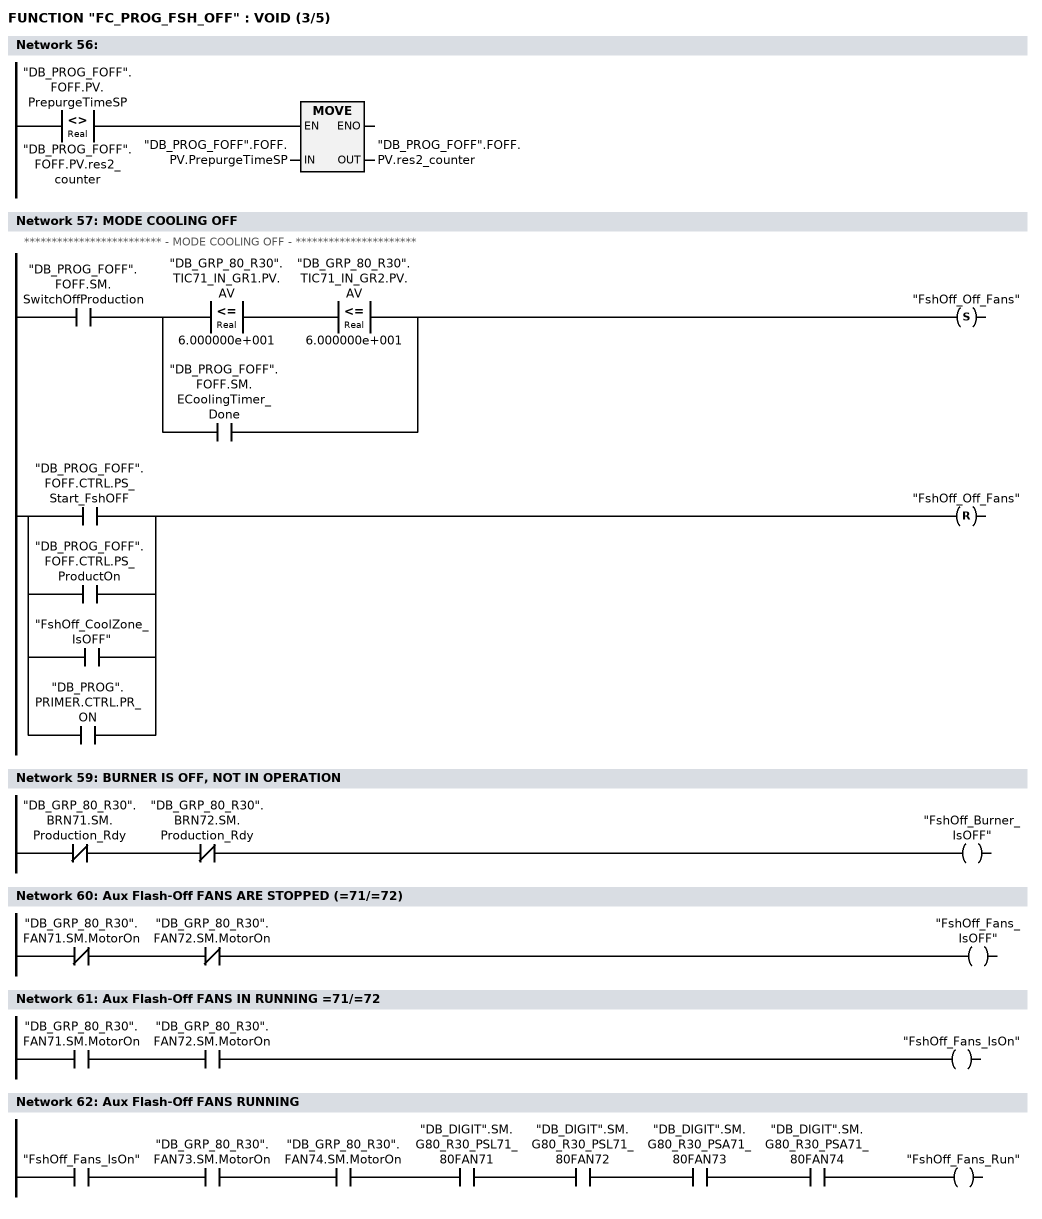
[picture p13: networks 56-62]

      U(    ;
      L     "DB_PROG_FOFF".FOFF.PV.PrepurgeTimeSP;
      L     "DB_PROG_FOFF".FOFF.PV.res2_counter;
      <>R   ;
      )     ;
      SPBNB _00b;
      L     "DB_PROG_FOFF".FOFF.PV.PrepurgeTimeSP;
      T     "DB_PROG_FOFF".FOFF.PV.res2_counter;
_00b: NOP   0;
NETWORK
TITLE =MODE COOLING OFF
//
//************************* - MODE COOLING OFF - **********************
//
      U     "DB_PROG_FOFF".FOFF.SM.SwitchOffProduction;
      U(    ;
      U(    ;
      L     "DB_GRP_80_R30".TIC71_IN_GR1.PV.AV;
      L     6.000000e+001;
      <=R   ;
      )     ;
      U(    ;
      L     "DB_GRP_80_R30".TIC71_IN_GR2.PV.AV;
      L     6.000000e+001;
      <=R   ;
      )     ;
      O     "DB_PROG_FOFF".FOFF.SM.ECoolingTimer_Done;
      )     ;
      S     "FshOff_Off_Fans";
      U(    ;
      O     "DB_PROG_FOFF".FOFF.CTRL.PS_Start_FshOFF;
      O     "DB_PROG_FOFF".FOFF.CTRL.PS_ProductOn;
      O     "FshOff_CoolZone_IsOFF";
      O     "DB_PROG".PRIMER.CTRL.PR_ON;
      )     ;
      R     "FshOff_Off_Fans";
      NOP   0;
NETWORK
TITLE =

NETWORK
TITLE =BURNER IS OFF, NOT IN OPERATION

      UN    "DB_GRP_80_R30".BRN71.SM.Production_Rdy;
      UN    "DB_GRP_80_R30".BRN72.SM.Production_Rdy;
      =     "FshOff_Burner_IsOFF";
NETWORK
TITLE =Aux Flash-Off FANS ARE STOPPED (=71/=72)

      UN    "DB_GRP_80_R30".FAN71.SM.MotorOn;
      UN    "DB_GRP_80_R30".FAN72.SM.MotorOn;
      =     "FshOff_Fans_IsOFF";
NETWORK
TITLE =Aux Flash-Off FANS IN RUNNING =71/=72

      U     "DB_GRP_80_R30".FAN71.SM.MotorOn;
      U     "DB_GRP_80_R30".FAN72.SM.MotorOn;
      =     "FshOff_Fans_IsOn";
NETWORK
TITLE =Aux Flash-Off FANS RUNNING

      U     "FshOff_Fans_IsOn";
      U     "DB_GRP_80_R30".FAN73.SM.MotorOn;
      U     "DB_GRP_80_R30".FAN74.SM.MotorOn;
      U     "DB_DIGIT".SM.G80_R30_PSL71_80FAN71;
      U     "DB_DIGIT".SM.G80_R30_PSL71_80FAN72;
      U     "DB_DIGIT".SM.G80_R30_PSA71_80FAN73;
      U     "DB_DIGIT".SM.G80_R30_PSA71_80FAN74;
      =     "FshOff_Fans_Run";
NETWORK
TITLE =COOLING ZONE FANS IS OFF (=73FAN01)
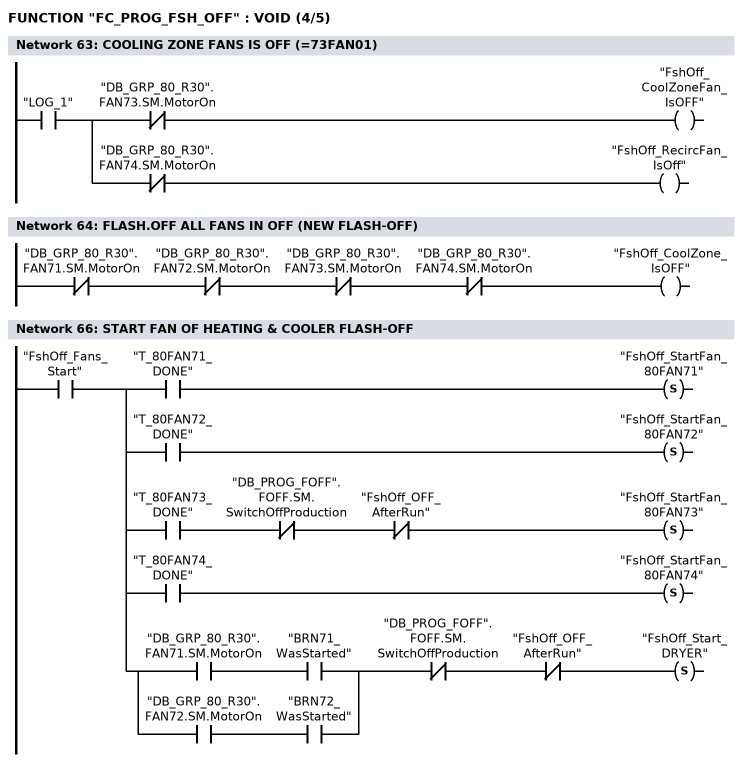
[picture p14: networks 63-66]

      U     "LOG_1";
      =     L      0.0;
      U     L      0.0;
      UN    "DB_GRP_80_R30".FAN73.SM.MotorOn;
      =     "FshOff_CoolZoneFan_IsOFF";
      U     L      0.0;
      UN    "DB_GRP_80_R30".FAN74.SM.MotorOn;
      =     "FshOff_RecircFan_IsOff";
NETWORK
TITLE =FLASH.OFF ALL FANS IN OFF (NEW FLASH-OFF)

      UN    "DB_GRP_80_R30".FAN71.SM.MotorOn;
      UN    "DB_GRP_80_R30".FAN72.SM.MotorOn;
      UN    "DB_GRP_80_R30".FAN73.SM.MotorOn;
      UN    "DB_GRP_80_R30".FAN74.SM.MotorOn;
      =     "FshOff_CoolZone_IsOFF";
NETWORK
TITLE =

NETWORK
TITLE =START FAN OF HEATING & COOLER FLASH-OFF

      U     "FshOff_Fans_Start";
      =     L      0.0;
      U     L      0.0;
      U     "T_80FAN71_DONE";
      S     "FshOff_StartFan_80FAN71";
      U     L      0.0;
      U     "T_80FAN72_DONE";
      S     "FshOff_StartFan_80FAN72";
      U     L      0.0;
      U     "T_80FAN73_DONE";
      UN    "DB_PROG_FOFF".FOFF.SM.SwitchOffProduction;
      UN    "FshOff_OFF_AfterRun";
      S     "FshOff_StartFan_80FAN73";
      U     L      0.0;
      U     "T_80FAN74_DONE";
      S     "FshOff_StartFan_80FAN74";
      U     L      0.0;
      U(    ;
      U     "DB_GRP_80_R30".FAN71.SM.MotorOn;
      U     "BRN71_WasStarted";
      O     ;
      U     "DB_GRP_80_R30".FAN72.SM.MotorOn;
      U     "BRN72_WasStarted";
      )     ;
      UN    "DB_PROG_FOFF".FOFF.SM.SwitchOffProduction;
      UN    "FshOff_OFF_AfterRun";
      S     "FshOff_Start_DRYER";
NETWORK
TITLE =RESET FAN OF HEATING FLASH-OFF AND COOLING FAN
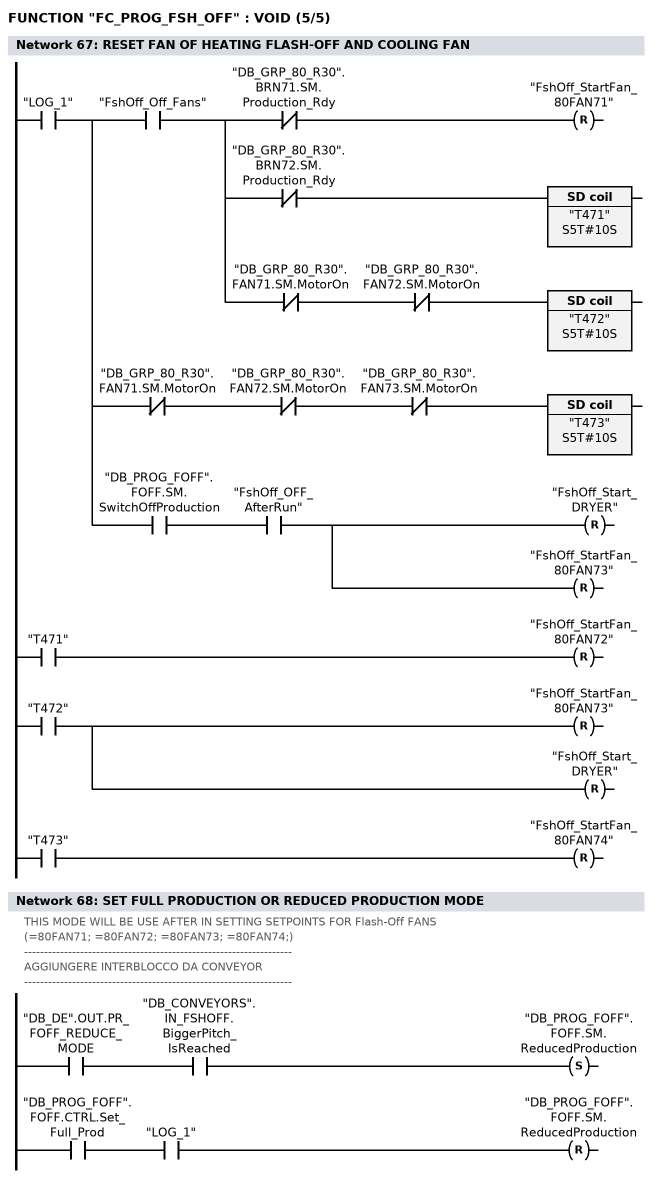
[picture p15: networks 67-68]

      U     "LOG_1";
      =     L      0.0;
      U     L      0.0;
      U     "FshOff_Off_Fans";
      =     L      0.1;
      U     L      0.1;
      UN    "DB_GRP_80_R30".BRN71.SM.Production_Rdy;
      R     "FshOff_StartFan_80FAN71";
      U     L      0.1;
      UN    "DB_GRP_80_R30".BRN72.SM.Production_Rdy;
      L     S5T#10S;
      SE    "T471";
      NOP   0;
      NOP   0;
      NOP   0;
      U     "T471";
      R     "FshOff_StartFan_80FAN72";
      U     L      0.1;
      UN    "DB_GRP_80_R30".FAN71.SM.MotorOn;
      UN    "DB_GRP_80_R30".FAN72.SM.MotorOn;
      L     S5T#10S;
      SE    "T472";
      NOP   0;
      NOP   0;
      NOP   0;
      U     "T472";
      R     "FshOff_StartFan_80FAN73";
      R     "FshOff_Start_DRYER";
      U     L      0.0;
      UN    "DB_GRP_80_R30".FAN71.SM.MotorOn;
      UN    "DB_GRP_80_R30".FAN72.SM.MotorOn;
      UN    "DB_GRP_80_R30".FAN73.SM.MotorOn;
      L     S5T#10S;
      SE    "T473";
      NOP   0;
      NOP   0;
      NOP   0;
      U     "T473";
      R     "FshOff_StartFan_80FAN74";
      U     L      0.0;
      U     "DB_PROG_FOFF".FOFF.SM.SwitchOffProduction;
      U     "FshOff_OFF_AfterRun";
      R     "FshOff_Start_DRYER";
      R     "FshOff_StartFan_80FAN73";
NETWORK
TITLE =SET FULL PRODUCTION OR REDUCED PRODUCTION MODE
//THIS MODE WILL BE USE AFTER IN SETTING SETPOINTS FOR Flash-Off FANS
//(=80FAN71; =80FAN72; =80FAN73; =80FAN74;)
//-------------------------------------------------------------------
//AGGIUNGERE INTERBLOCCO DA CONVEYOR
//-------------------------------------------------------------------
      U     "DB_DE".OUT.PR_FOFF_REDUCE_MODE;
      U     "DB_CONVEYORS".IN_FSHOFF.BiggerPitch_IsReached;
      S     "DB_PROG_FOFF".FOFF.SM.ReducedProduction;
      U     "DB_PROG_FOFF".FOFF.CTRL.Set_Full_Prod;
      U     "LOG_1";
      R     "DB_PROG_FOFF".FOFF.SM.ReducedProduction;
      NOP   0;
NETWORK
TITLE =

NETWORK
TITLE =********** END CYCLE OF Flash-Off *************



END_FUNCTION

